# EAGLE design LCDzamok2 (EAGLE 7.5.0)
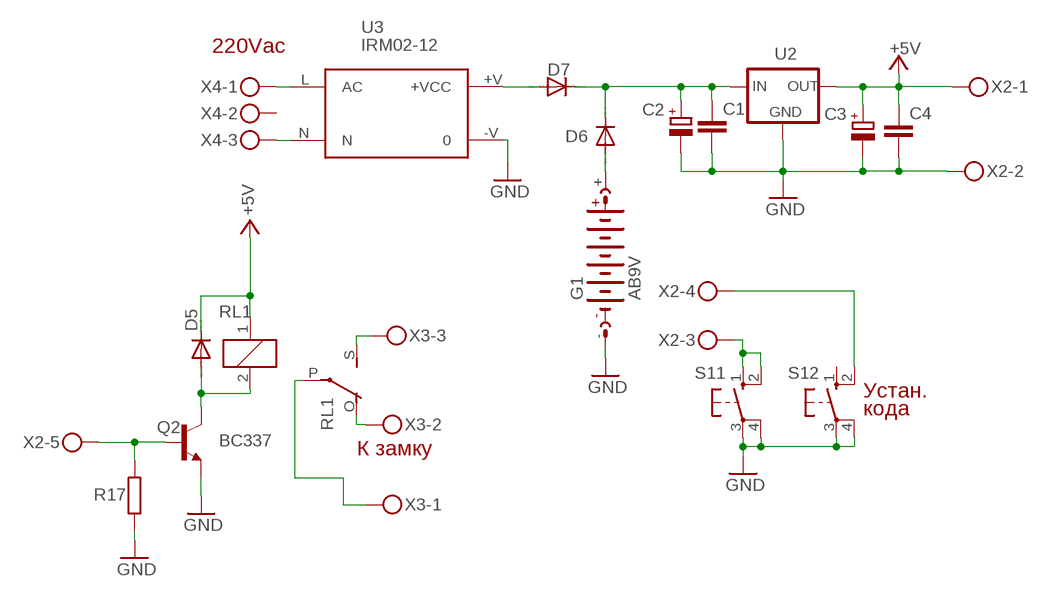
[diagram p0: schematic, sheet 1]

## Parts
C1  C-EUC1206  [C1206]
C2  CPOL-EUE5-8.5  [E5-8,5]
C3  CPOL-EUE5-8.5  [E5-8,5]
C4  C-EUC1206  [C1206]
D5  1N4004  [DO41-10]
D6  1N4004  [DO41-10]
D7  1N4004  [DO41-10]
G1  AB9V  [AB9V]
Q2  BC337  [TO92]
R17  R-EU_0204/7  [0204/7]
RL1  G5LE  [G5LE]
S11  40-XX  [B3F-40XX]
S12  40-XX  [B3F-40XX]
U2  78XXL  [78XXL]
U3  IRM02-12  IRM02  [IRM02]
X2  MKDSN1,5/5-5,08  [MKDSN1,5/5-5,08]
X3  MKDSN1,5/3-5,08  [MKDSN1,5/3-5,08]
X4  MKDSN1,5/3-5,08  [MKDSN1,5/3-5,08]

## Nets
+5V: C3.+ C4.1 D5.C RL1.1 U2.OUT X2.1
GND: C1.2 C2.- C3.- C4.2 G1.- Q2.1(E) R17.1 S11.3(P) S11.4(P1) S12.3(P) S12.4(P1) U2.GND U3.-V X2.2
N$1: RL1.O(2:O) X3.2
N$2: RL1.S(2:S) X3.3
N$3: S12.2(S1) X2.4
N$4: RL1.P(2:P) X3.1
N$6: Q2.2(B) R17.2 X2.5
N$7: S11.1(S) S11.2(S1) X2.3
N$8: C1.1 C2.+ D6.C D7.C U2.IN
N$9: U3.L(AC) X4.1
N$10: U3.N X4.3
N$11: D7.A U3.+V(+VCC)
N$12: D6.A G1.+
Q1: D5.A Q2.3(C) RL1.2
Unconnected: S12.1(S) X4.2

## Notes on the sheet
- 220Vac
- Устан.
- кода
- К замку

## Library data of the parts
C1 C4 = rcl:C-EU: CAPACITOR, European symbol
C2 C3 = rcl:CPOL-EU: POLARIZED CAPACITOR, European symbol
D5-D7 = diode:1N4004: DIODE
G1 = battery:AB9V: 9-V BATTERY CLIP
Q2 = transistor:BC337: NPN TRANSISTOR
R17 = rcl:R-EU_: RESISTOR, European symbol
RL1 = relay:G5LE: RELAY 1 x switch, 10 A/120 V AC, 8 A/30 V DC, Omron; OC_FARNELL: unknown; OC_NEWARK: unknown
S11 S12 = switch-omron:40-XX: OMRON SWITCH; MF: OMRON COMPONENTS USA; MPN: B3F-4000; OC_FARNELL: 176434; OC_NEWARK: 36K3105
U2 = v-reg:78XXL: VOLTAGE REGULATOR
U3 = acdc:IRM02: 2W Single Output ACDC converter
X2 = con-phoenix-508:MKDSN1,5/5-5,08: MKDSN 1,5/ 5-5,08 Printklemme Nennstrom: 13,5 A Nennspannung: 250 V Rastermaß: 5,08 mm Polzahl: 5 Anschlussart: Schraubanschluss Montage: Löten Anschlussrichtung Leiter/Platine: 0 ° Artikelnummer: 1729157 Source: http://eshop.phoenixcontact.com .. 1729157.pdf
X3 X4 = con-phoenix-508:MKDSN1,5/3-5,08: MKDSN 1,5/ 3-5,08 Printklemme Nennstrom: 13,5 A Nennspannung: 250 V Rastermaß: 5,08 mm Polzahl: 3 Anschlussart: Schraubanschluss Montage: Löten Anschlussrichtung Leiter/Platine: 0 ° Artikelnummer: 1729131 Source: http://eshop.phoenixcontact.com .. 1729131.pdf

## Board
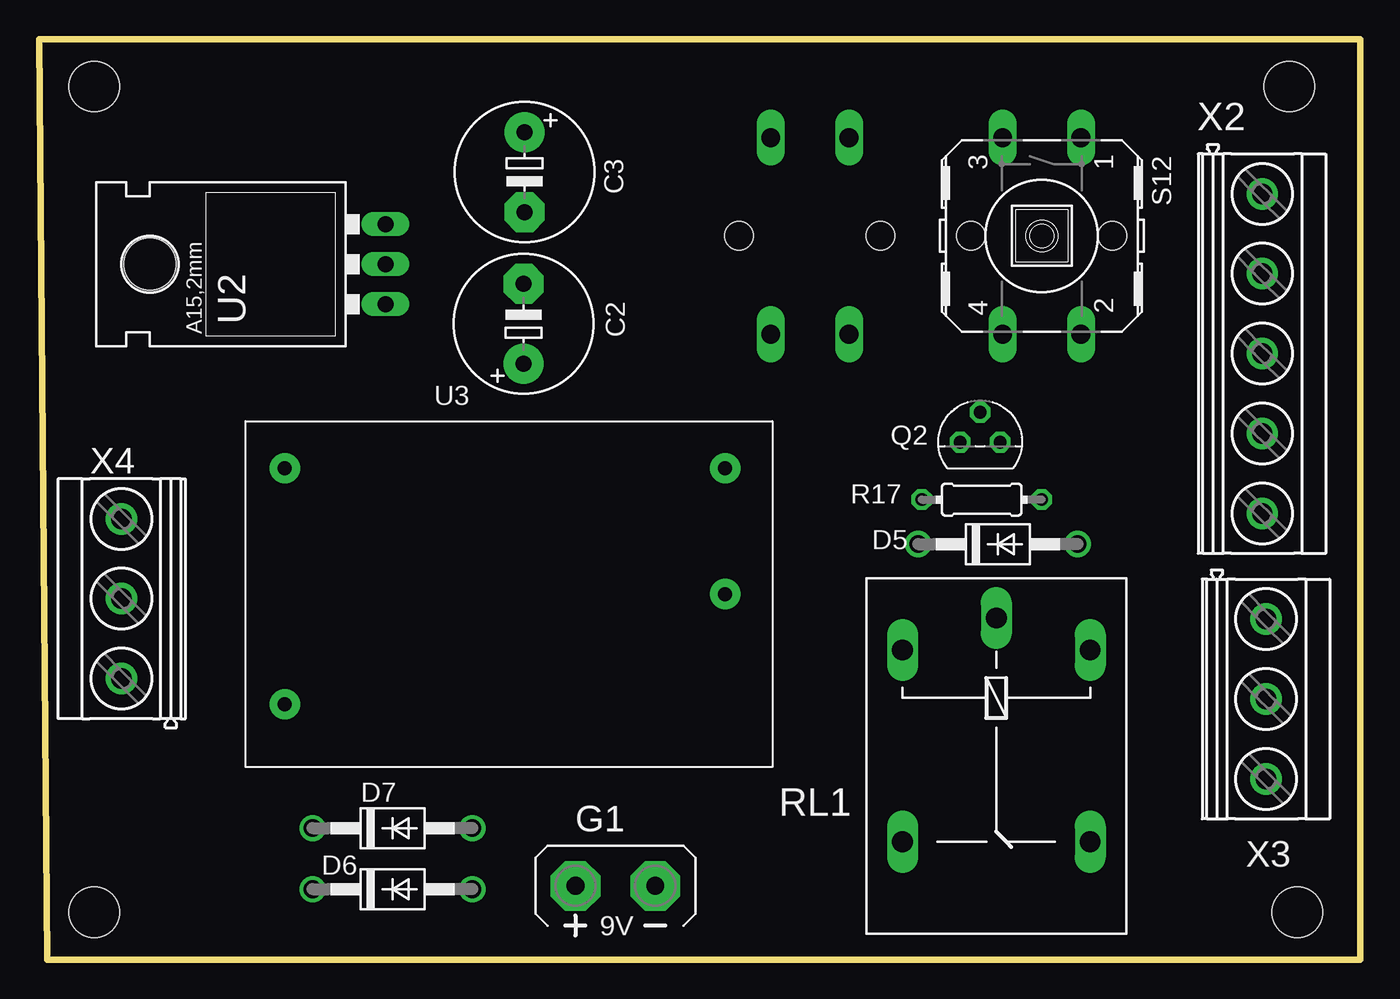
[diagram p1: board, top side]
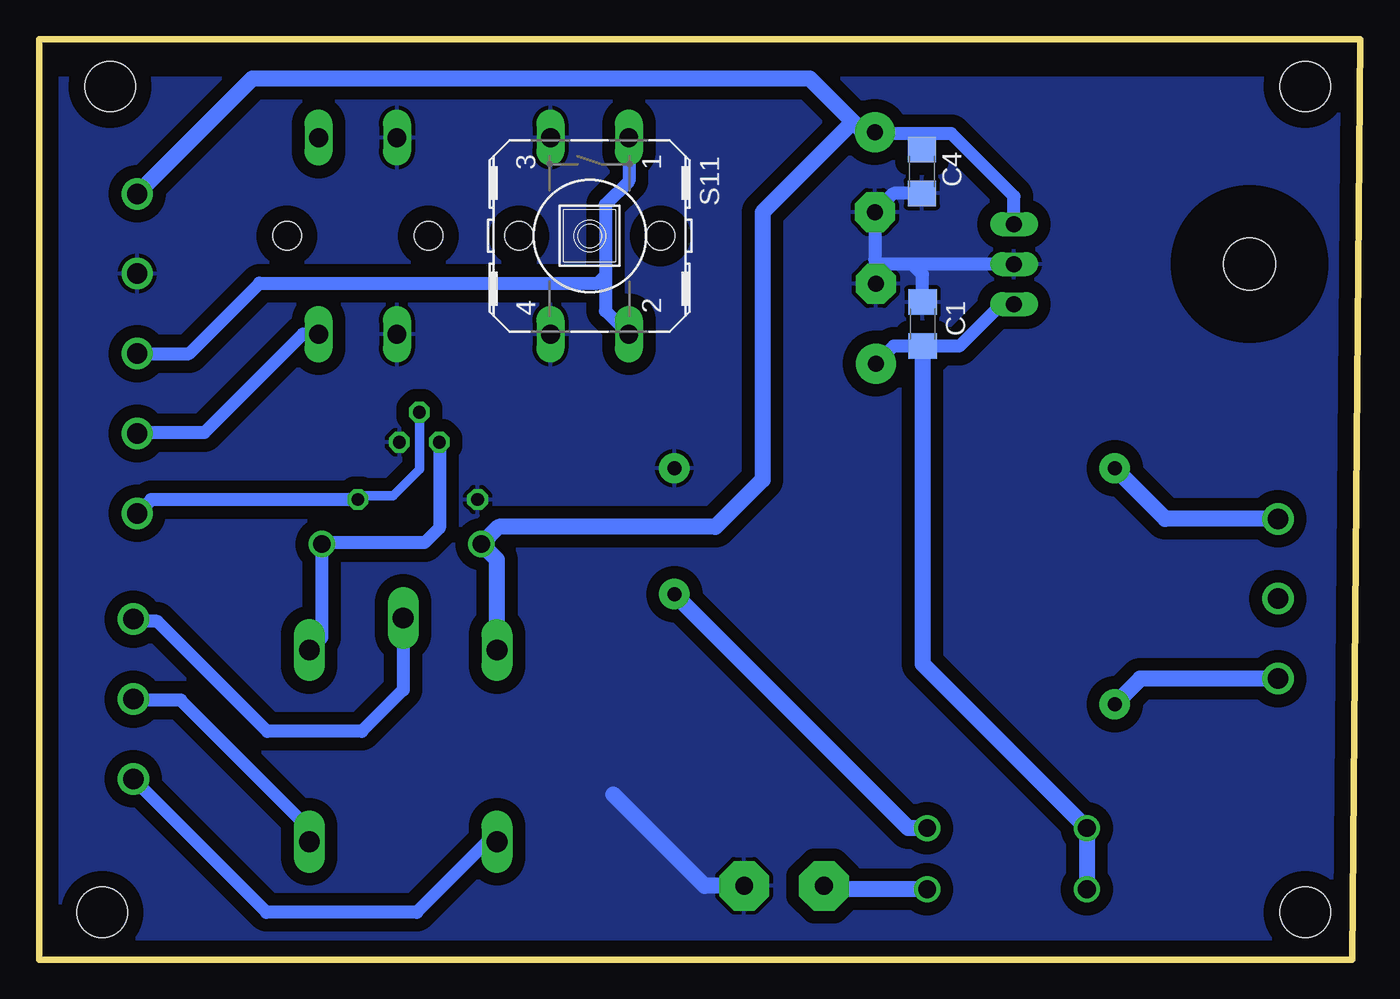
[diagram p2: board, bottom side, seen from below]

Size 84 x 58.5 mm. Coordinates in mm from the lower left corner, seen from the top.
Outline: 0.5,0 0,58.5 84,58.5 84,0 0.5,0
Copper layers (1*16): Top 0.035mm / dielectric 1.5mm / Bottom 0.035mm
Design rules "default": minimum track width 10mil, minimum drill 24mil, track to track 8mil, track to pad 8mil, pad to pad 8mil, via to via 8mil, smd to smd 8mil, copper to edge 40mil, drill to drill 8mil, minimum pad ring 10mil, minimum via ring 8mil, stop-mask expansion 4mil, vias tented up to drill 0mil, thermal gap 10mil
Holes 3.2 mm at 3.5,3 3.5,55.5 79.5,55.5 80,3

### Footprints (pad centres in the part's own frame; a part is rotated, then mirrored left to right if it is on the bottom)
C1206 = smd 1.6 x 1.8: 1 -1.4,0; 2 1.4,0
E5-8,5 = drill 1.016 pad 2.54: + -2.54,0 | drill 1.016 pad 2.54 octagon: - 2.54,0
DO41-10 = drill 1.118: A 5.08,0; C -5.08,0
AB9V = drill 1.118 pad 3.15 octagon: + 0,2.54; - 0,-2.54
TO92 = drill 0.813 octagon: 1 1.27,0; 2 0,1.905; 3 -1.27,0
0204/7 = drill 0.813 octagon: 1 -3.81,0; 2 3.81,0
G5LE = drill 1.321 long: 1 -7.493,-5.969; 2 -7.493,5.969; O 4.699,5.969; P -9.525,0; S 4.699,-5.969
B3F-40XX = drill 1.194 long: 1 -6.248,2.489; 2 6.248,2.489; 3 -6.248,-2.489; 4 6.248,-2.489 | hole 1.803: 0,-4.496; 0,4.496
78XXL = drill 1.016 long: GND 0,-3.81; IN -2.54,-3.81; OUT 2.54,-3.81 | hole 3.302: 0,11.176
IRM02 = drill 0.9 pad 1.93: +V 30.5,-11; -V 30.5,-3; L 2.5,-18; N 2.5,-3
MKDSN1,5/5-5,08 = drill 1.3 pad 2: 1 -10.181,0.025; 2 -5.101,0.025; 3 -0.021,0.025; 4 5.059,0.025; 5 10.139,0.025
MKDSN1,5/3-5,08 = drill 1.3 pad 2: 1 -7.641,0.025; 2 -2.561,0.025; 3 2.519,0.025

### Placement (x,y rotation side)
C1  27.83,40.4 90 bottom
C2  30.8,40.42 90 top
C3  30.86,50.06 270 top
C4  27.87,50.1 270 bottom
D5  60.96,26.41 0 top
D6  22.46,4.47 0 top
D7  22.46,8.35 0 top
G1  36.64,4.69 90 top
Q2  59.83,32.89 0 top
R17  59.93,29.24 0 top
RL1  60.86,12.19 270 top
S11  49,46 270 bottom
S12  63.75,46 270 top
U2  18.21,44.21 90 top
U3  13.11,34.23 0 top
X2  77.75,38.5 270 top
X3  78,14 270 top
X4  5.25,25.5 90 top

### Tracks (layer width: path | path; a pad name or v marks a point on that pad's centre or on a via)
+5V
  Bottom 0.813: U2.OUT 22.02,48.52 26,52.5 27.5,52.5 | 27.5,52.5 30.76,52.5 C3.+ | C4.1 27.87,52.13 27.5,52.5
  Bottom 1.016: C3.+ 31.6,52.6 32.25,53.25 | 32.25,53.25 35,56 70.46,56 X2.1 | RL1.1 54.89,25.42 D5.C 54.79,27.5 41,27.5 38,30.5 38,47.5 32.25,53.25
GND
  Bottom 0.813: C4.2 29.68,48.7 C3.- 30.86,44.5 | 30.86,44.5 30.86,43.02 C2.- | U2.GND 28.5,44.21 | 28.5,44.21 30.57,44.21 30.86,44.5 | C1.2 27.83,43.54 28.5,44.21
  Bottom 1.016: G1.- 41.69,4.69 47.5,10.5
  pour Bottom (isolate 0.813): 1.5,56 83.5,56 83.5,0.5 1,0.5 1,56
N$1
  Bottom 0.813: RL1.O 66.83,8.33 75,16.5 77.96,16.5 X3.2
N$2
  Bottom 0.813: RL1.S 55.51,7.49 60,3 69.54,3 X3.3
N$3
  Bottom 0.813: S12.2 67.25,39.75 73.5,33.5 77.72,33.5 X2.4
N$4
  Bottom 0.813: RL1.P 60.86,17.14 63.5,14.5 69.5,14.5 76.5,21.5 77.88,21.5 X3.1
N$6
  Bottom 0.61: Q2.2 59.83,31.17 61.5,29.5 63.48,29.5 R17.2
  Bottom 0.813: R17.2 76.9,29.24 X2.5
N$7
  Bottom 0.813: S11.1 46.51,49.49 48,48 48,43.5 | 48,43.5 48,41.24 S11.2 | X2.3 74.48,38.52 70,43 48.5,43 48,43.5
N$8
  Bottom 0.813: U2.IN 22.83,41.67 25.5,39 C1.1 29.68,39 C2.+
  Bottom 1.016: C1.1 27.83,18.8 D7.C D6.C
N$9
  Bottom 1.016: X4.1 13.98,17.86 U3.L
N$10
  Bottom 1.016: X4.3 12.4,28.02 U3.N
N$11
  Bottom 1.016: D7.A 28.73,8.35 U3.+V
N$12
  Bottom 1.016: D6.A 33.88,4.47 G1.+
Q1
  Bottom 0.813: RL1.2 66.04,20.47 D5.A 65.95,26.5 59.5,26.5 58.56,27.44 Q2.3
